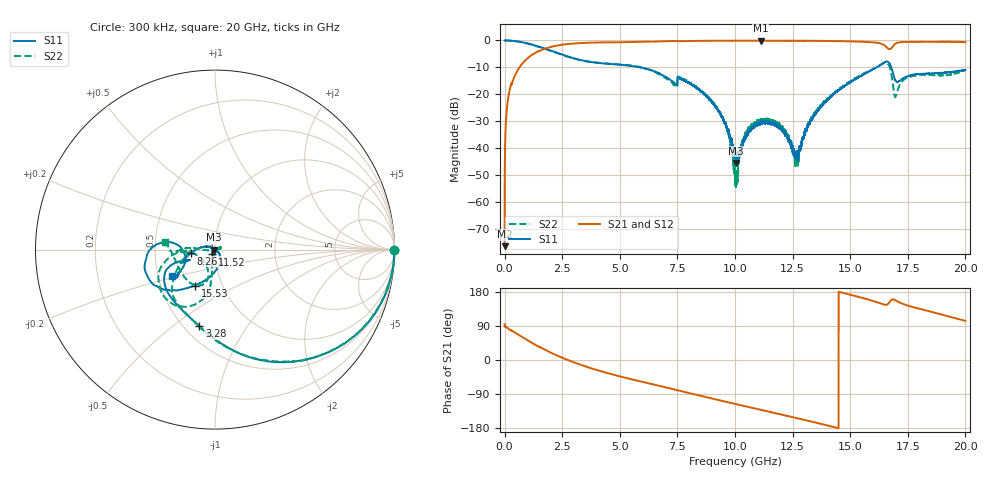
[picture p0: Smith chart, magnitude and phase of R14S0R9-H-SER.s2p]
!{R14S0R9}
!Johanson Technology Inc.
!www.johansontechnology.com
!Test Board Conditions:
!Substrate Type  RO4350B
!Substrate Thickness  20 mil
!Substrate Dk  3.66
!TL Type: GCPW
!TL Trace Width  36 mil
!TL Gap  12 mil
!Electrode orientation  Horizontal
!DUT TOPOLOGY	SERIES
!Mounting Pad LxW  26x36 mil
! Created Wed Nov 25 17:33:21 2020
! 2 Port Network Data from SP1.SP block
! freq  magS11  angS11  magS21  angS21  magS12  angS12  magS22  angS22
# khz S ma R 50
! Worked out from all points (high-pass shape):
!   20001 points, 300 kHz to 20 GHz, reference 50 ohm
!   highest |S21| = -0.08 dB at 11.12 GHz (marker M1); lowest = -76.3 dB at 300 kHz (marker M2)
!   |S21| within 3 dB of the highest: 1.75 GHz to 16.65 GHz (14.9 GHz wide, 162 % of centre); 16.76 GHz to end of sweep
!   lowest |S11| = -45.4 dB at 10.05 GHz (marker M3), VSWR 1.01, Z = 49.5 - j0.122 ohm
!   |S11| at or under -10 dB: 5.887849 GHz to 5.888531 GHz (681.9 kHz wide, 0.0116 % of centre); 5.89 GHz to 16.13 GHz (10.24 GHz wide, 93 % of centre); 16.78 GHz to end of sweep
!   |S22| runs from -54.4 to 0.0 dB; largest |S21 - S12| = 0.014
!   S11 on the Smith chart (normalised r, x): 300 kHz: open; 3.28 GHz: 0.59, -0.63; 8.261 GHz: 0.76, -0.03; 11.52 GHz: 0.97, -0.05; 15.53 GHz: 0.74, -0.31; 20 GHz: 0.59, -0.19
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300  0.9956 -0.2  0.0001532 94.6  0.0002277 87.6  0.9971 -0.2
134300  0.9963 -5.6  0.074 84.2  0.07449 84.1  0.997 -5.6
514300  0.9661 -19.7  0.2549 70.0  0.2555 70.1  0.965 -19.7
1600300  0.7416 -57.6  0.6627 31.9  0.6641 31.9  0.7348 -57.9
3280300  0.4356 -101.5  0.8925 -12.1  0.8932 -12.2  0.4337 -102.6
3334300  0.43 -102.7  0.895 -13.3  0.8953 -13.3  0.4277 -103.7
6667300  0.2493 -161.0  0.9602 -67.5  0.9603 -67.4  0.2432 -151.7
8261300  0.1376 -171.1  0.9794 -90.9  0.9802 -90.8  0.1426 175.8
9528300  0.03134 154.0  0.9874 -109.2  0.9891 -109.1  0.0313 -171.6
1.00003e7  0.008235 -174.9  0.9883 -115.8  0.9881 -115.8  0.002481 -144.7
1.00453e7  0.005353 -166.7  0.9875 -116.5  0.988 -116.4  0.002441 -69.0
1.04003e7  0.01521 -95.3  0.9887 -121.5  0.988 -121.4  0.01537 6.3
1.11183e7  0.03053 -108.8  0.9907 -131.5  0.9865 -131.5  0.03466 16.0
1.15163e7  0.03083 -119.0  0.9874 -137.1  0.9859 -137.0  0.03311 19.5
1.21233e7  0.01978 -136.1  0.9882 -145.4  0.9857 -145.5  0.02163 22.3
1.26743e7  0.008125 -73.1  0.985 -153.3  0.9851 -153.2  0.007066 -51.5
1.33343e7  0.03479 -44.7  0.9819 -162.7  0.9844 -162.7  0.03662 -109.4
1.55343e7  0.2293 -119.0  0.945 163.7  0.9512 163.6  0.2345 -99.0
1.66673e7  0.3905 -171.3  0.6962 149.6  0.6875 149.9  0.3541 -152.9
1.69783e7  0.1776 -177.2  0.8797 157.1  0.8791 157.3  0.09218 -129.2
1.75823e7  0.2229 -148.8  0.9378 142.1  0.9422 142.1  0.2121 -111.1
2e7  0.2836 -148.6  0.9318 103.2  0.9212 103.1  0.2828 171.9
